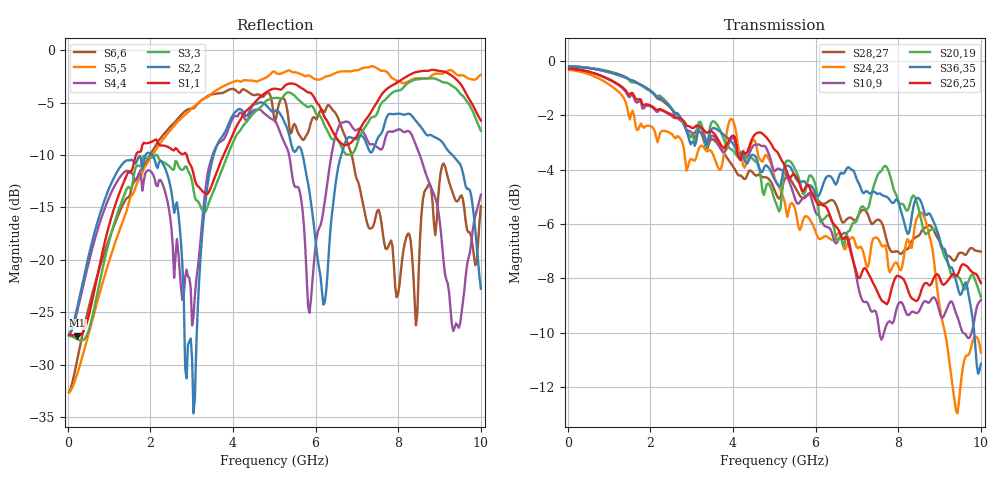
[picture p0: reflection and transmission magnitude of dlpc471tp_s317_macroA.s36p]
! Touchstone(R) file created by SIwave 2018.1.0
! Touchstone(R) file created on Mon Dec 10 15:08:10 2018
! Port[1] = DCLK_AN_DIE_207
! Port[2] = DCLK_AN_LGA_A4
! Port[3] = DCLK_AP_DIE_206
! Port[4] = DCLK_AP_LGA_A3
! Port[5] = D_AN_0__DIE_226
! Port[6] = D_AN_0__LGA_A7
! Port[7] = D_AN_1__DIE_222
! Port[8] = D_AN_1__LGA_C2
! Port[9] = D_AN_2__DIE_218
! Port[10] = D_AN_2__LGA_A5
! Port[11] = D_AN_3__DIE_212
! Port[12] = D_AN_3__LGA_A9
! Port[13] = D_AN_4__DIE_202
! Port[14] = D_AN_4__LGA_E1
! Port[15] = D_AN_5__DIE_196
! Port[16] = D_AN_5__LGA_E3
! Port[17] = D_AN_6__DIE_192
! Port[18] = D_AN_6__LGA_G3
! Port[19] = D_AN_7__DIE_188
! Port[20] = D_AN_7__LGA_A11
! Port[21] = D_AP_0__DIE_225
! Port[22] = D_AP_0__LGA_A8
! Port[23] = D_AP_1__DIE_221
! Port[24] = D_AP_1__LGA_B2
! Port[25] = D_AP_2__DIE_217
! Port[26] = D_AP_2__LGA_A6
! Port[27] = D_AP_3__DIE_211
! Port[28] = D_AP_3__LGA_A10
! Port[29] = D_AP_4__DIE_201
! Port[30] = D_AP_4__LGA_D1
! Port[31] = D_AP_5__DIE_195
! Port[32] = D_AP_5__LGA_D3
! Port[33] = D_AP_6__DIE_191
! Port[34] = D_AP_6__LGA_F3
! Port[35] = D_AP_7__DIE_187
! Port[36] = D_AP_7__LGA_A12
! S-parameters
# Hz S MA R 50.000000
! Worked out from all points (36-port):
!   299 points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, 33.44 MHz to 10 GHz, reference 50 ohm
!   strongest paths, dB at 33.44 MHz, 2.508 GHz, 5.017 GHz, 7.525 GHz, 10 GHz:
!     S26,25: -0.3, -2.0, -3.3, -8.6, -8.2
!     S36,35: -0.2, -1.8, -4.4, -4.9, -11.1
!     S20,19: -0.2, -1.7, -5.2, -4.1, -8.7
!     S10,9: -0.3, -2.0, -4.1, -9.8, -8.8
!     S24,23: -0.3, -2.7, -4.4, -6.6, -10.7
!     S28,27: -0.2, -1.8, -4.8, -5.8, -7.0
!   lowest |S11| = -27.3 dB at 234.1 MHz (marker M1), VSWR 1.09, Z = 54.1 + j1.9 ohm
!   |S11| at or under -10 dB: start of sweep to 1.654 GHz; 2.88 GHz to 3.774 GHz (893.7 MHz wide, 26.9 % of centre)
